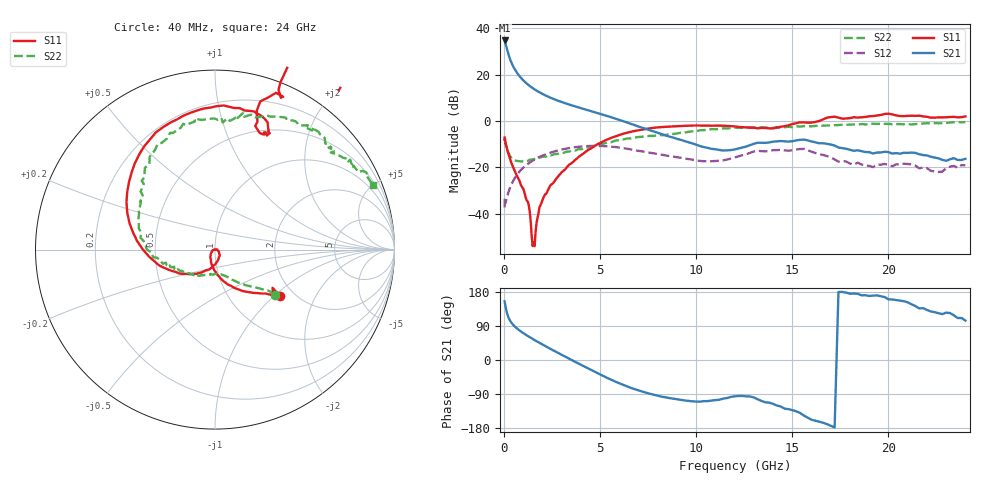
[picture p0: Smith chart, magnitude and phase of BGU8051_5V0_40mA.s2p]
! BGU8051_5V0_40mA
! Date/time Tue Jun 16 11:03:17 2015
! VAR V_out= 5.0000
! VAR I_out= 39.9900
! VAR V_in= 4.5950
! VAR I_in= 0.5319
# MHz S MA R 50
!  Freq-MHz  S11-mag  S11-arg  S21-mag  S21-arg  S12-mag  S12-arg  S22-mag  S22-arg
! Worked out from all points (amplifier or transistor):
!   187 points, 40 MHz to 24 GHz, reference 50 ohm
!   highest |S21| = 34.8 dB at 40 MHz (marker M1)
!   |S21| within 3 dB of that: start of sweep to 138.5 MHz
!   unconditionally stable (mu >= 1): 480.8 MHz to 14.06 GHz
!   at 750 MHz: K = 1.02, MAG = 20.5 dB, |S12| = -22.4 dB
!   at 5.4 GHz: K = 1.20, MAG = 3.8 dB, |S12| = -10.9 dB
!   at 24 GHz: K = -1.00, MSG = 1.4 dB, |S12| = -19.1 dB
!   lowest NFmin = 0.35 dB at 400 MHz
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40  0.4416 -35.5  54.64 154.7  0.01369 32.1  0.4179 -37.3
60  0.4121 -38.2  51.41 149.2  0.02185 39.9  0.3738 -37.6
80  0.3582 -43.1  47.54 143.5  0.01717 39.2  0.3307 -40.9
120  0.301 -51.9  41.3 133.1  0.01975 45.7  0.2824 -46.2
160  0.2578 -59.4  35.69 124.6  0.02262 48.4  0.2495 -50.8
200  0.2214 -65.9  31.05 118.0  0.02549 51.7  0.2234 -55.0
220  0.2082 -69.6  29.15 115.1  0.02779 53.5  0.2147 -56.2
280  0.1716 -76.9  24.28 107.9  0.03289 56.4  0.1903 -61.1
360  0.1365 -85.8  19.71 100.9  0.04005 59.3  0.1671 -65.4
440  0.1106 -92.8  16.51 95.4  0.0473 60.4  0.1549 -70.4
550  0.08677 -101.8  13.48 89.2  0.05734 60.5  0.1426 -75.2
750  0.05857 -113.5  10.06 80.5  0.07555 59.1  0.1376 -83.6
950  0.03794 -129.9  8.012 73.0  0.0936 56.4  0.1348 -90.6
1550  0.002411 105.1  4.965 54.0  0.1446 45.5  0.1502 -110.8
2600  0.04789 -63.5  2.974 24.6  0.2197 23.2  0.1919 -134.4
4100  0.1938 -134.9  1.85 -15.1  0.2845 -10.2  0.2505 -157.0
5600  0.4364 173.8  1.2 -52.4  0.2798 -42.6  0.3509 -177.3
8200  0.7419 112.6  0.5253 -96.8  0.1883 -76.6  0.4964 147.3
12200  0.7476 66.7  0.2565 -94.9  0.1738 -74.1  0.7134 103.2
16200  0.9581 68.3  0.348 -160.2  0.2047 -149.7  0.7872 70.5
20200  1.39 34.6  0.1993 159.7  0.1059 -160.6  0.8522 43.9
24000  1.257 21.6  0.1534 104.0  0.1108 -178.9  0.9525 22.1
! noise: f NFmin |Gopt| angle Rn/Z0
400  0.3511  0.1066  41.24  0.0482
550  0.3563  0.09263  53.09  0.049
950  0.3832  0.07665  93.14  0.0503
1250  0.4159  0.08416  121.5  0.0506
1600  0.4678  0.1041  144.9  0.0508
1900  0.5239  0.1246  158.9  0.0511
2250  0.6029  0.1497  171.3  0.0521
2600  0.6967  0.1753  181.3  0.0543
3300  0.9281  0.2277  197  0.0641
4000  1.218  0.2816  208.8  0.0844
